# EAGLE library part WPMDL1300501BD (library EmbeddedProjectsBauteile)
MagI³C-FDRM Fixed Step Down Regulator 5V 3A
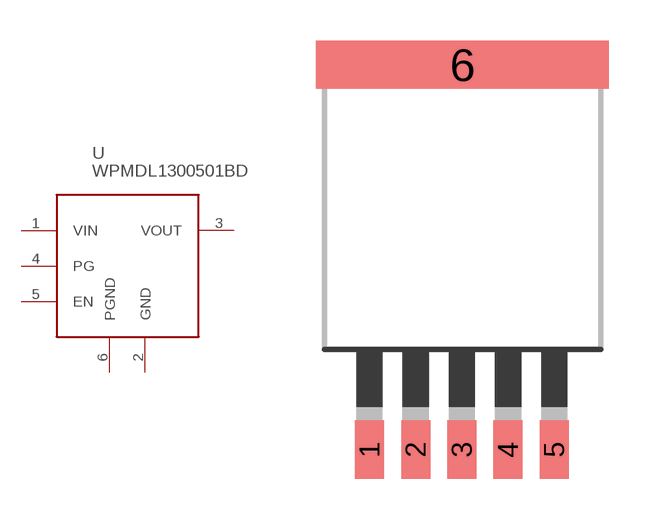
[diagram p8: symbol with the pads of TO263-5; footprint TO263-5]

Designator prefix -

## WPMDL1300501BD (EP: 401014)  [TO263-5]
1  VIN  in
2  GND  pas
3  VOUT  out
4  PG  out
5  EN  in
6  PGND  pas

## Footprint TO263-5 (pad centres in mm)
smd 1.067 x 2.159: 1 -3.424,-9.109; 2 -1.722,-9.109; 3 -0.02,-9.109; 4 1.682,-9.109; 5 3.384,-9.109
smd 10.8 x 1.778: 6 0,5.08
